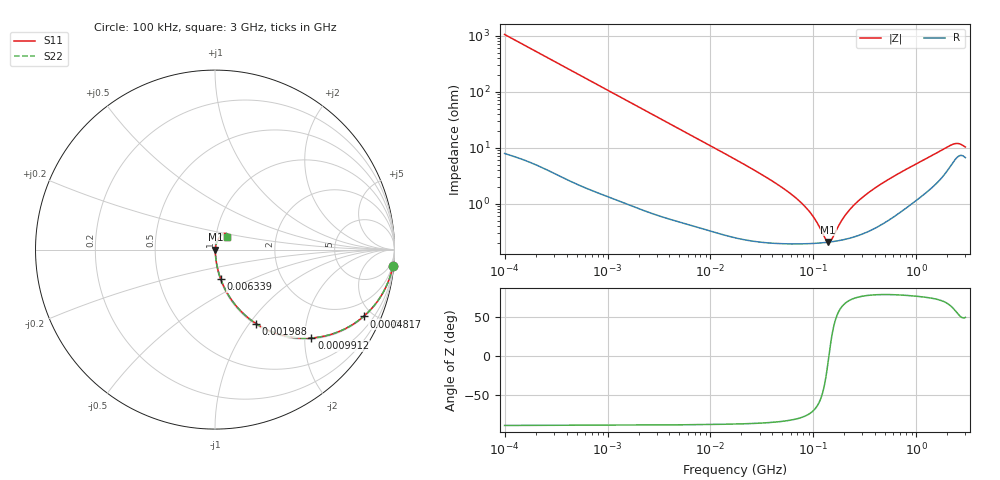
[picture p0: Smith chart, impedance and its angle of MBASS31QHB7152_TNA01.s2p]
! MBASS31QHB7152_TNA01  S-PARAMETER MODEL  ( Standard Model )
! Model Generated by TAIYO YUDEN Corporation (http://www.ty-top.com)
! Version 1.0
! TAIYO YUDEN Control No. 220601
! Copyright(c) 2013 TAIYO YUDEN CO.,LTD. All Rights Reserved.
! Product Description (link to TY-COMPAS)
! https://ds.yuden.co.jp/TYCOMPAS/or/detail?pn=MBASS31QHB7152KTNA01&u=M
! Products Name : Multilayer Ceramic Capacitors
! Characteristics :
!  Capacitance : 1500 [pF] , Rated Voltage : 630 [V] , TCC : X7R
!  Case Size : 3.2 x 1.6 / 0.126 x 0.063 [mm/inch] , Thickness : 1.15 / 0.045 [mm/inch]
!  (Conditions: Temperature = 25 [degC] , DC Bias Voltage = 0 [V])
! External Node Assignments :
!  1  o---| |---o  2
! GND o---------o GND
! Frequency Range : 100kHz  -  3GHz  [ 401 STEP ]
# MHZ S RI R 50
! Freq[MHz].  S11 Real  S11 Imag  S21 Real  S21 Imag  S12 Real  S12 Imag  S22 Real  S22 Imag
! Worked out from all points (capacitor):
!   401 points, 100 kHz to 3 GHz, reference 50 ohm
!   read as one part in series: C = 1.51 nF near 105.3 kHz
!   lowest |Z| = 207 mohm at 139.7 MHz (marker M1)
!   series resonance near 141.6 MHz, so ESL is about 840 pH
!   S11 on the Smith chart (normalised r, x): 100 kHz: 1, -21; 481.7 kHz: 1.05, -4.42; 991.2 kHz: 1.03, -2.16; 1.988 MHz: 1.02, -1.08; 6.339 MHz: 1.01, -0.34; 3 GHz: 1.13, +0.16
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0.1  0.9904 -0.0938  0.0096 0.0938  0.0096 0.0938  0.9904 -0.0938
0.252895  0.9443 -0.2246  0.0557 0.2246  0.0557 0.2246  0.9443 -0.2246
0.481683  0.8276 -0.3725  0.1724 0.3725  0.1724 0.3725  0.8276 -0.3725
0.562235  0.7799 -0.409  0.2201 0.409  0.2201 0.409  0.7799 -0.409
0.991196  0.5376 -0.4924  0.4624 0.4924  0.4624 0.4924  0.5376 -0.4924
1.987766  0.2298 -0.4131  0.7702 0.4131  0.7702 0.4131  0.2298 -0.4131
3.161081  0.1086 -0.3023  0.8914 0.3023  0.8914 0.3023  0.1086 -0.3023
6.3393  0.0322 -0.1648  0.9678 0.1648  0.9678 0.1648  0.0322 -0.1648
17.7727  0.0061 -0.0603  0.9939 0.0603  0.9939 0.0603  0.0061 -0.0603
55.23785  0.00221 -0.0168  0.9978 0.0168  0.9978 0.0168  0.00221 -0.0168
77.22239  0.00202 -0.00999  0.998 0.00999  0.998 0.00999  0.00202 -0.00999
97.38194  0.00199 -0.00594  0.998 0.00594  0.998 0.00594  0.00199 -0.00594
129.3002  0.00203 -0.00141  0.998 0.00141  0.998 0.00141  0.00203 -0.00141
139.694  0.00206 -0.000207  0.9979 0.000207  0.9979 0.000207  0.00206 -0.000207
150.9232  0.0021 0.000991  0.9979 -0.000991  0.9979 -0.000991  0.0021 0.000991
195.2919  0.0023 0.00506  0.9977 -0.00506  0.9977 -0.00506  0.0023 0.00506
246.2744  0.00262 0.00897  0.9974 -0.00897  0.9974 -0.00897  0.00262 0.00897
344.2911  0.00345 0.0155  0.9966 -0.0155  0.9966 -0.0155  0.00345 0.0155
547.5153  0.00589 0.0271  0.9941 -0.0271  0.9941 -0.0271  0.00589 0.0271
2145.926  0.0534 0.0906  0.9466 -0.0906  0.9466 -0.0906  0.0534 0.0906
2504.792  0.0715 0.0855  0.9285 -0.0855  0.9285 -0.0855  0.0715 0.0855
3000  0.0676 0.0689  0.9324 -0.0689  0.9324 -0.0689  0.0676 0.0689
